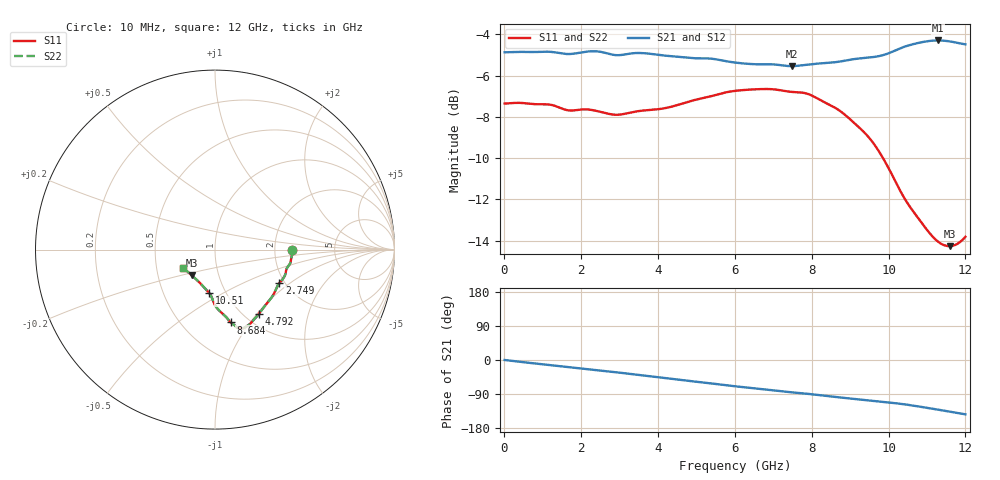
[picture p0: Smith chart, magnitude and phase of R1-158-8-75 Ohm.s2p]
!version-1
!date-10.2020
!Series
#GHZ	S	RI	R	50.0
!FREQ.GHZ	S11RE	S11IM	S21RE	S21IM	S12RE	S12IM	S22RE	S22IM
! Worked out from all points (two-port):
!   500 points, 10 MHz to 12 GHz, reference 50 ohm
!   highest |S21| = -4.29 dB at 11.28 GHz (marker M1); lowest = -5.5 dB at 7.483 GHz (marker M2)
!   |S21| within 3 dB of the highest: start of sweep to end of sweep
!   lowest |S11| = -14.3 dB at 11.59 GHz (marker M3), VSWR 1.48, Z = 37.1 - j11.1 ohm
!   |S11| at or under -10 dB: 9.857 GHz to end of sweep
!   |S22| runs from -14.3 to -6.6 dB; largest |S21 - S12| = 0
!   S11 on the Smith chart (normalised r, x): 10 MHz: 2.50, +0.00; 2.749 GHz: 1.88, -0.84; 4.792 GHz: 1.17, -1.03; 8.684 GHz: 0.83, -0.81; 10.51 GHz: 0.84, -0.43; 12 GHz: 0.69, -0.15
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0.01  0.4288 0  0.571 -0.0003  0.571 -0.0003  0.4288 0
1.09126  0.422 -0.0666  0.5602 -0.1198  0.5602 -0.1198  0.422 -0.0666
1.66794  0.399 -0.1064  0.5352 -0.1823  0.5352 -0.1823  0.399 -0.1064
2.02836  0.3935 -0.1321  0.5281 -0.2173  0.5281 -0.2173  0.3935 -0.1321
2.34072  0.381 -0.1588  0.5159 -0.2525  0.5159 -0.2525  0.381 -0.1588
2.7492  0.3588 -0.1866  0.4864 -0.288  0.4864 -0.288  0.3588 -0.1866
3.44601  0.3264 -0.2492  0.4428 -0.3569  0.4428 -0.3569  0.3264 -0.2492
4.02269  0.2907 -0.2973  0.3928 -0.4031  0.3928 -0.4031  0.2907 -0.2973
4.79158  0.2466 -0.3563  0.3176 -0.4535  0.3176 -0.4535  0.2466 -0.3563
5.44034  0.2122 -0.3949  0.2548 -0.4878  0.2548 -0.4878  0.2122 -0.3949
6.01701  0.1852 -0.4217  0.1892 -0.5047  0.1892 -0.5047  0.1852 -0.4217
6.83397  0.1574 -0.4378  0.1077 -0.5231  0.1077 -0.5231  0.1574 -0.4378
7.48273  0.1379 -0.4365  0.0429 -0.5269  0.0429 -0.5269  0.1379 -0.4365
8.01134  0.1197 -0.432  -0.00535 -0.5345  -0.00535 -0.5345  0.1197 -0.432
8.68413  0.0869 -0.4056  -0.0782 -0.5356  -0.0782 -0.5356  0.0869 -0.4056
9.47705  0.0383 -0.354  -0.1598 -0.5306  -0.1598 -0.5306  0.0383 -0.354
10.0057  -0.00553 -0.2985  -0.2135 -0.5265  -0.2135 -0.5265  -0.00553 -0.2985
10.5103  -0.0316 -0.2426  -0.2817 -0.5217  -0.2817 -0.5217  -0.0316 -0.2426
10.9187  -0.0643 -0.2071  -0.3457 -0.497  -0.3457 -0.497  -0.0643 -0.2071
11.2792  -0.0963 -0.1739  -0.3992 -0.4613  -0.3992 -0.4613  -0.0963 -0.1739
11.5915  -0.1292 -0.1441  -0.4387 -0.4193  -0.4387 -0.4193  -0.1292 -0.1441
12  -0.1767 -0.1018  -0.4789 -0.3561  -0.4789 -0.3561  -0.1767 -0.1018
